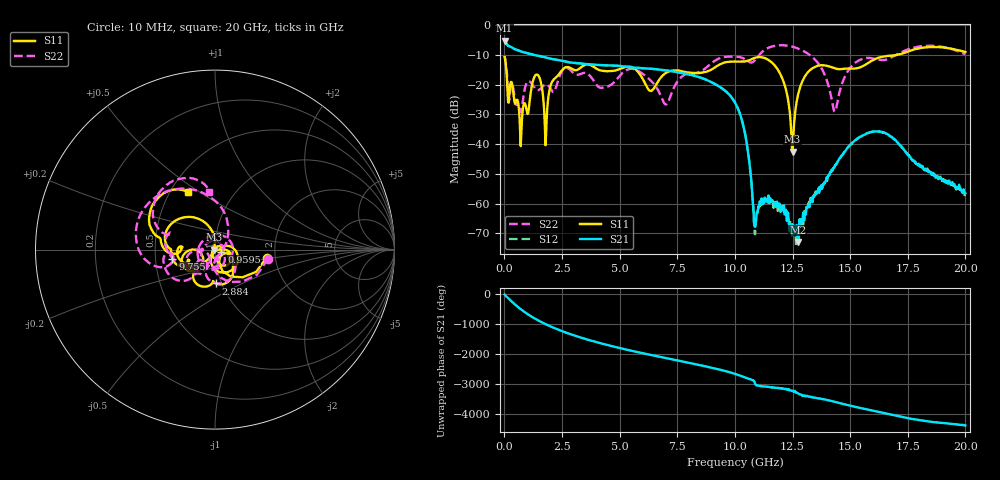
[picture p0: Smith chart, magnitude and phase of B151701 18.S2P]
!  2-Port S-parameters saved by WinCal
! VAR MeasName=S-Parameters (CALIBRATED_DATA) read from VNA (N5244A)
! VAR MeasDate=2015-12-24 19:10:17
! VAR NAME=B151701 18
! VAR FILENAME=B151701 18.S2P
! VAR DATE=2015-12-24 19:10:17
! VAR PHYS_PORTS=1,3
# Hz S DB R 50
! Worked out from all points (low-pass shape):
!   801 points, 10 MHz to 20 GHz, reference 50 ohm
!   highest |S21| = -5.17 dB at 10 MHz (marker M1); lowest = -72.9 dB at 12.73 GHz (marker M2)
!   |S21| within 3 dB of the highest: start of sweep to 485.8 MHz
!   lowest |S11| = -42.5 dB at 12.5 GHz (marker M3), VSWR 1.02, Z = 49.3 - j0.0479 ohm
!   |S11| at or under -10 dB: start of sweep to 17.05 GHz
!   |S22| runs from -29.2 to -6.8 dB; largest |S21 - S12| = 0.0013
!   S11 on the Smith chart (normalised r, x): 10 MHz: 1.79, -0.18; 959.5 MHz: 1.07, -0.03; 2.884 GHz: 0.94, -0.37; 9.755 GHz: 0.61, -0.07; 20 GHz: 0.61, +0.45
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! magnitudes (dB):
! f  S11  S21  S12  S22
! 10 MHz  -10.7  -5.2  -5.2  -10.4
! 634.7 MHz  -28.5  -8.6  -8.6  -27.1
! 959.5 MHz  -28.3  -9.3  -9.3  -19.5
! 1.434 GHz  -16.6  -10.3  -10.3  -21.8
! 1.809 GHz  -36.7  -10.9  -10.9  -20.0
! 2.084 GHz  -18.9  -11.4  -11.4  -22.3
! 2.884 GHz  -14.5  -12.6  -12.6  -15.3
! 3.358 GHz  -14.0  -12.9  -12.9  -16.2
! 5.607 GHz  -14.4  -14.2  -14.2  -14.8
! 6.682 GHz  -18.8  -14.9  -14.9  -22.1
! 9.755 GHz  -12.3  -23.4  -23.4  -10.6
! 10.01 GHz  -12.2  -26.1  -26.1  -10.6
! 10.48 GHz  -12.2  -38.1  -38.0  -11.7
! 10.88 GHz  -11.0  -67.8  -70.3  -11.7
! 11.95 GHz  -16.2  -60.8  -61.4  -6.8
! 12.5 GHz  -42.5  -66.9  -68.0  -7.3
! 12.73 GHz  -23.8  -72.9  -71.5  -7.8
! 13.35 GHz  -14.6  -59.5  -57.9  -10.7
! 14.33 GHz  -14.5  -47.4  -47.6  -29.0
! 15.15 GHz  -14.6  -39.2  -39.2  -13.1
! 16.68 GHz  -10.3  -37.0  -36.9  -11.3
! 20 GHz  -9.0  -56.5  -57.1  -9.9
